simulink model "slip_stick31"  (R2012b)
settings: Solver=ode2  StartTime=0.0  StopTime=100  FixedStep=0.001  MaxStep=0.001  RelTol=1e-3
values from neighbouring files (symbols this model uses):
  c = 2200    [coulomb_1.m]    (also in coulomb_10.m = 0.1; coulomb_11.m = 0; coulomb_2.m; coulomb_3.m)
  k = 10    [coulomb_10.m]    (also in coulomb_11.m; diff_filter_1.m = 250; diff_filter_2.m = 250; dry_friction_1.m = 2200)
  m = 400    [coulomb_1.m]    (also in coulomb_10.m = 10; coulomb_11.m = 10; coulomb_2.m; coulomb_3.m)
  vb = 0.1    [coulomb_10.m]    (also in coulomb_11.m; slip_stick_3.m; slip_stick_31.m; slip_stick_3_1.m)

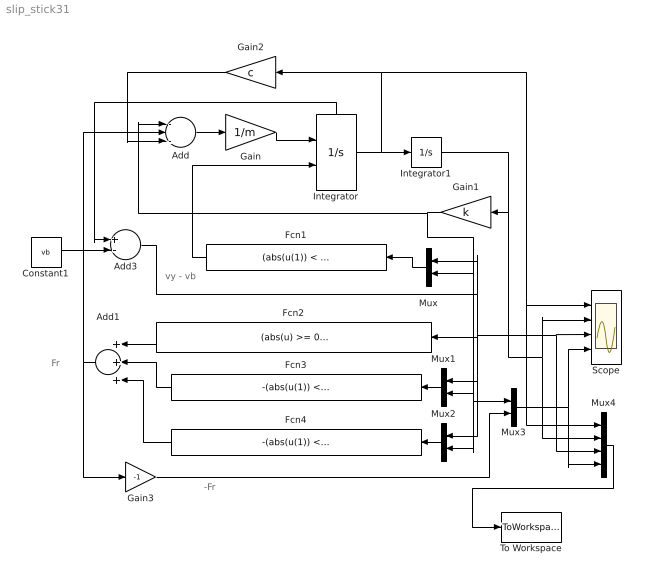
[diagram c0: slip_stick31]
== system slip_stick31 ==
  note: -Fr
  note: vy - vb
  note: Fr
  Add : Sum  Inputs=---
  Add1 : Sum  Inputs=+++
  Add3 : Sum  Inputs=+-
  Constant1 : Constant  Value=vb
  Fcn1 : Fcn  Expr=(abs(u(1)) < 0.001)*(abs(u(2)) < FH)
  Fcn2 : Fcn  Expr=(abs(u) >= 0.001)*(FG + (FH-FG)*exp(-(u/vs)^2))*sgn(u)
  Fcn3 : Fcn  Expr=-(abs(u(1)) < 0.001)*(abs(u(2)) >= FH)*FH*sgn(u(2))
  Fcn4 : Fcn  Expr=-(abs(u(1)) < 0.001)*(abs(u(2)) < FH)*u(2)
  Gain : Gain  Gain=1/m
  Gain1 : Gain  Gain=k
  Gain2 : Gain  Gain=c
  Gain3 : Gain  Gain=-1
  Integrator : Integrator  ExternalReset=level  InitialCondition=vb  ShowStatePort=on
  Integrator1 : Integrator
  Mux{,1..3} (4 alike) : Mux  Inputs=2
  Mux4 : Mux
  Scope : Scope  NumInputPorts=4
  To Workspace : ToWorkspace  VariableName=y  SampleTime=-1  SaveFormat=Structure With Time
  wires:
  Add/1 -> Gain/1
  Gain/1 -> Integrator/1
  Integrator1/1 -> Mux4/2, Scope/2, Gain1/1
  Gain2/1 -> Add/3
  Constant1/1 -> Add3/2
  Add3/1 -> Mux4/3, Scope/3, Fcn2/1, Mux2/1, Mux1/1, Mux/1
  Integrator/1 -> Integrator1/1, Mux4/1, Scope/1, Gain2/1
  Integrator/State -> Add3/1
  Mux/1 -> Fcn1/1
  Fcn1/1 -> Integrator/2
  Fcn2/1 -> Add1/1
  Add1/1 -> Gain3/1, Add/2
  Fcn3/1 -> Add1/2
  Mux1/1 -> Fcn3/1
  Gain1/1 -> Mux3/1, Mux2/2, Mux1/2, Mux/2, Add/1
  Mux2/1 -> Fcn4/1
  Fcn4/1 -> Add1/3
  Mux3/1 -> Mux4/4, Scope/4
  Gain3/1 -> Mux3/2
  Mux4/1 -> To Workspace/1
